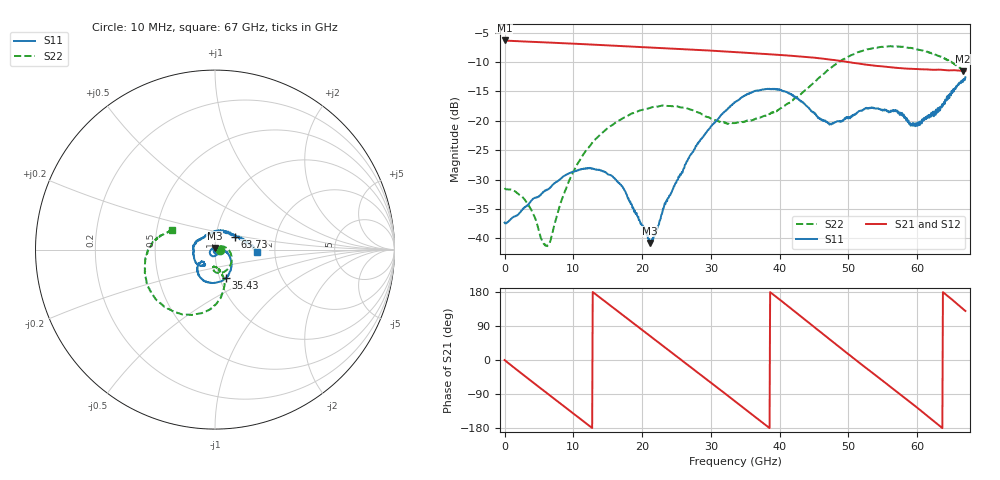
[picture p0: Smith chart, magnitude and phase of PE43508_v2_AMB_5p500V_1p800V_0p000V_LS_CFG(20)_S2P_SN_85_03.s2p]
!Keysight Technologies,N5227A,US51270237,A.10.43.00
!Date: Wednesday, August 22, 2018 17:08:37
!Correction: S11(Full 2 Port(1,3))
!S31(Full 2 Port(1,3))
!S13(Full 2 Port(1,3))
!S33(Full 2 Port(1,3))
!S2P File: Measurements: S11, S31, S13, S33:
# Hz S  dB  R 50
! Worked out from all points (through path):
!   801 points, 10 MHz to 67 GHz, reference 50 ohm
!   highest |S21| = -6.34 dB at 10 MHz (marker M1); lowest = -11.5 dB at 66.67 GHz (marker M2)
!   group delay of S21, straight-line fit = 39.2 ps
!   lowest |S11| = -40.8 dB at 21.11 GHz (marker M3), VSWR 1.02, Z = 49.9 + j0.907 ohm
!   |S11| at or under -10 dB: start of sweep to end of sweep
!   |S22| runs from -41.3 to -7.3 dB; largest |S21 - S12| = 0.0033
!   S11 on the Smith chart (normalised r, x): 10 MHz: 1.03, -0.00; 35.43 GHz: 1.07, -0.35; 63.73 GHz: 1.24, +0.18; 67 GHz: 1.61, -0.04
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1e7  -37.33 -1.8  -6.34 -0.2  -6.34 -0.2  -31.43 -1.8
3.02455e9  -34.70 -30.0  -6.52 -43.5  -6.52 -43.5  -33.59 -30.5
6.206575e9  -31.76 -59.8  -6.68 -88.3  -6.68 -88.2  -41.33 6.1
8.7187e9  -29.34 -84.0  -6.82 -123.4  -6.81 -123.4  -32.22 38.9
1.123082e10  -28.19 -106.2  -6.96 -158.4  -6.95 -158.4  -26.17 20.5
1.391042e10  -28.43 -132.0  -7.11 164.3  -7.10 164.3  -22.36 -1.4
1.684124e10  -30.83 -164.0  -7.28 123.5  -7.27 123.6  -19.83 -24.7
2.111185e10  -40.80 95.3  -7.53 64.3  -7.52 64.3  -17.83 -55.6
2.236791e10  -37.80 42.1  -7.60 46.8  -7.60 46.8  -17.55 -64.2
2.722469e10  -25.56 -7.1  -7.89 -20.8  -7.89 -20.8  -18.16 -90.4
3.049045e10  -20.33 -27.9  -8.11 -66.6  -8.10 -66.5  -19.86 -96.9
3.3505e10  -16.86 -52.9  -8.32 -108.9  -8.31 -108.8  -20.40 -90.8
3.543096e10  -15.38 -68.4  -8.46 -136.0  -8.46 -135.9  -19.99 -84.7
3.970158e10  -14.60 -108.0  -8.79 163.6  -8.78 163.7  -18.19 -77.9
4.472582e10  -18.41 -139.2  -9.23 91.4  -9.21 91.5  -13.79 -75.0
4.732169e10  -20.56 -131.8  -9.60 53.8  -9.58 53.7  -11.10 -84.5
5.016876e10  -19.53 -125.4  -10.05 12.8  -10.05 12.8  -8.96 -100.4
5.586291e10  -18.59 -175.9  -10.86 -67.4  -10.87 -67.7  -7.34 -138.8
5.979858e10  -20.44 115.1  -11.20 -123.0  -11.22 -123.2  -7.82 -164.1
6.373424e10  -17.47 32.4  -11.35 179.0  -11.43 178.9  -9.21 172.5
6.666505e10  -13.37 0.6  -11.52 134.5  -11.59 134.9  -11.32 157.6
6.7e10  -12.61 -2.9  -11.51 129.3  -11.58 129.6  -11.53 155.1
